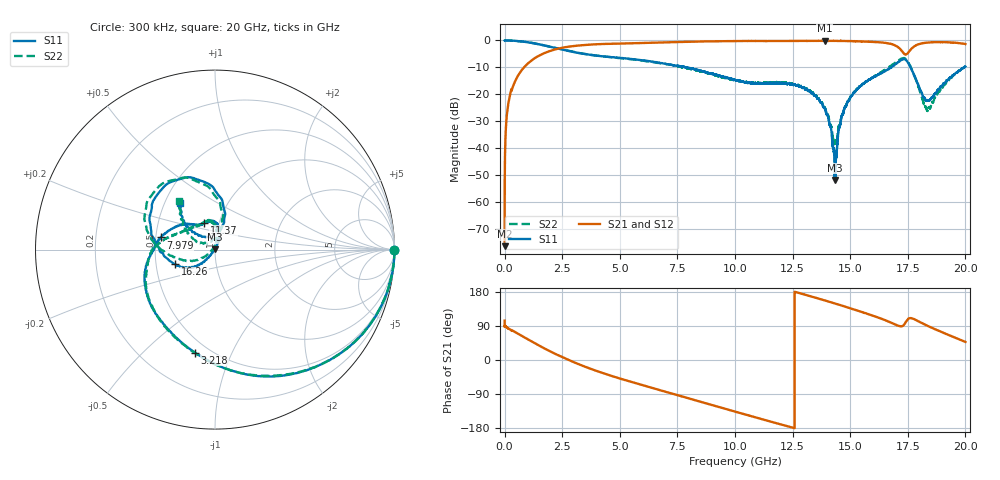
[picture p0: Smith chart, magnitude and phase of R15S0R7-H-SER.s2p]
!{R15S0R7}
!Johanson Technology Inc.
!www.johansontechnology.com
!Test Board Conditions:
!Substrate Type  RO4350B
!Substrate Thickness  20 mil
!Substrate Dk  3.66
!TL Type: GCPW
!TL Trace Width  34 mil
!TL Gap  10 mil
!Electrode orientation  Horizontal
!DUT TOPOLOGY	SERIES
!Mounting Pad LxW  26x52 mil
! Created Sat Feb  6 12:07:54 2021
# hz S ma R 50
! 2 Port Network Data from SP1.SP block
! freq  magS11  angS11  magS21  angS21  magS12  angS12  magS22  angS22
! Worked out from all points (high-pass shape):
!   20001 points, 300 kHz to 20 GHz, reference 50 ohm
!   highest |S21| = -0.13 dB at 13.89 GHz (marker M1); lowest = -76.4 dB at 300 kHz (marker M2)
!   |S21| within 3 dB of the highest: 2.287 GHz to 17.17 GHz (14.88 GHz wide, 153 % of centre); 17.65 GHz to end of sweep
!   lowest |S11| = -51.8 dB at 14.34 GHz (marker M3), VSWR 1.01, Z = 49.8 + j0.11 ohm
!   |S11| at or under -10 dB: 7.903 GHz to 16.79 GHz (8.887 GHz wide, 72 % of centre); 16.79001 GHz to 16.79356 GHz (3.548 MHz wide, 0.0211 % of centre); 17.62 GHz to 19.94 GHz (2.325 GHz wide, 12.4 % of centre)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
!   |S22| runs from -38.5 to 0.0 dB; largest |S21 - S12| = 0.016
!   S11 on the Smith chart (normalised r, x): 300 kHz: open; 3.218 GHz: 0.42, -0.73; 7.979 GHz: 0.53, +0.08; 11.37 GHz: 0.85, +0.26; 16.26 GHz: 0.63, -0.11; 20 GHz: 0.60, +0.35
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300000  0.9954 -0.1  0.0001509 103.6  0.0001552 113.3  0.9955 -0.2
1.013e8  0.9989 -3.9  0.0426 85.9  0.04283 85.9  0.9988 -3.9
1.353e8  0.9981 -5.1  0.05678 84.6  0.0572 84.6  0.998 -5.1
5.113e8  0.9802 -17.9  0.1953 71.7  0.1957 71.9  0.9791 -17.9
1.6793e9  0.817 -57.9  0.5695 32.1  0.5711 32.1  0.8161 -57.6
3.2183e9  0.5849 -100.9  0.8052 -11.1  0.8062 -11.2  0.5858 -101.0
3.3343e9  0.574 -103.7  0.8138 -14.0  0.8152 -14.0  0.5744 -103.8
6.6673e9  0.3878 -168.2  0.914 -78.3  0.915 -78.2  0.3822 -168.4
7.9793e9  0.3109 167.4  0.9458 -101.0  0.9475 -101.0  0.3017 171.3
1.00003e10  0.1858 131.1  0.975 -136.1  0.976 -136.2  0.184 139.7
1.13723e10  0.1594 111.8  0.9761 -159.6  0.9778 -159.8  0.1635 110.0
1.33343e10  0.1054 75.0  0.9821 167.2  0.9799 167.2  0.1052 84.0
1.38863e10  0.05562 68.3  0.9856 157.3  0.9797 157.4  0.05647 78.3
1.43393e10  0.002574 154.6  0.9801 149.1  0.9811 149.1  0.01271 143.9
1.45823e10  0.03007 -133.2  0.9798 144.5  0.9782 144.5  0.0308 -149.8
1.49353e10  0.07634 -131.3  0.9743 137.9  0.9747 137.9  0.0779 -145.1
1.62613e10  0.235 -159.8  0.9232 111.0  0.9219 110.9  0.2421 -171.6
1.66673e10  0.2935 -176.5  0.8826 101.3  0.8675 101.3  0.3156 177.6
1.74293e10  0.4313 111.1  0.5503 101.7  0.5473 101.7  0.4427 116.9
1.77653e10  0.2299 77.6  0.7684 108.2  0.7636 108.1  0.2321 81.9
1.83843e10  0.07723 109.7  0.9161 89.3  0.9156 89.3  0.05308 123.8
2e10  0.3251 126.5  0.8603 47.7  0.8549 47.5  0.3343 126.3
